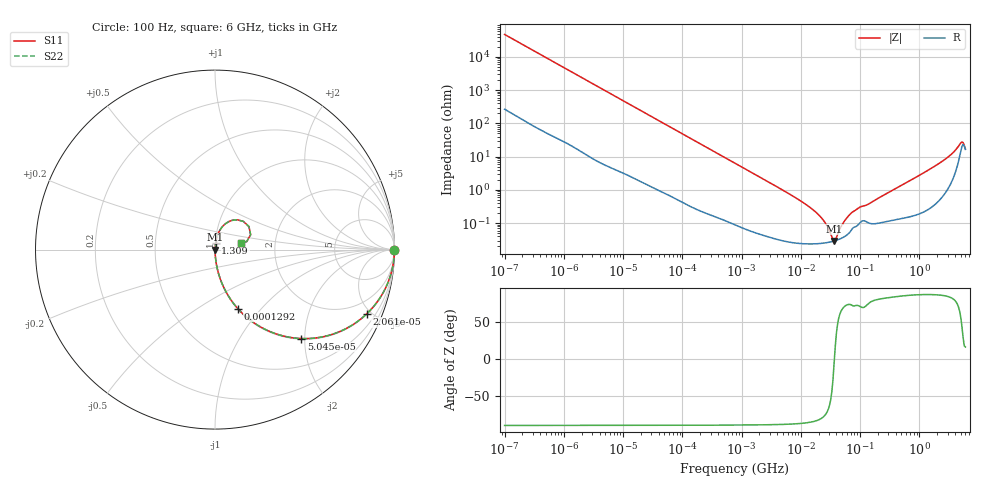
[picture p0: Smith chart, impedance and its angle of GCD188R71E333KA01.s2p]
!Murata Part Number: GCD188R71E333KA01
!These Parameters are Measured in Series Mode Connection
!Data Generated on Mar 13, 2026
!  o--ll--o
!Port1  Port2
!  o------o
!Operation Temp=25[degC], DC Bias Voltage=0[V]
!Freq. Start=100[Hz] Stop=6[GHz] 401[Steps]
# Hz S RI R 50
!Freq.(Hz) S11(Real) S11(Imag) S21(Real) S21(Imag) S12(Real) S12(Imag) S22(Real) S22(Imag)
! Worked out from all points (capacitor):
!   401 points, 100 Hz to 6 GHz, reference 50 ohm
!   read as one part in series: C = 33.5 nF near 109 Hz
!   lowest |Z| = 29.4 mohm at 36.42 MHz (marker M1)
!   series resonance near 36.95 MHz, so ESL is about 550 pH
!   S11 on the Smith chart (normalised r, x): 100 Hz: open; 20.61 kHz: 1.03, -4.69; 50.45 kHz: 1.02, -1.92; 129.2 kHz: 1.01, -0.75; 1.309 GHz: 1.00, +0.07; 6 GHz: 1.33, +0.09
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100  1 -0.00211  1.64e-05 0.00211  1.64e-05 0.00211  1 -0.00211
2008  0.998 -0.0418  0.002 0.0418  0.002 0.0418  0.998 -0.0418
7036  0.9782 -0.143  0.0218 0.143  0.0218 0.143  0.9782 -0.143
20606  0.8443 -0.359  0.1557 0.359  0.1557 0.359  0.8443 -0.359
40335  0.5901 -0.4878  0.4099 0.4878  0.4099 0.4878  0.5901 -0.4878
50455  0.4806 -0.4955  0.5194 0.4955  0.5194 0.4955  0.4806 -0.4955
129199  0.1269 -0.3284  0.8731 0.3284  0.8731 0.3284  0.1269 -0.3284
302498  0.0272 -0.1572  0.9728 0.1572  0.9728 0.1572  0.0272 -0.1572
774597  0.00491 -0.0633  0.9951 0.0633  0.9951 0.0633  0.00491 -0.0633
6353432  0.000329 -0.00764  0.9997 0.00764  0.9997 0.00764  0.000329 -0.00764
1.555665e7  0.000246 -0.00265  0.9998 0.00265  0.9998 0.00265  0.000246 -0.00265
2.434276e7  0.000254 -0.00117  0.9997 0.00117  0.9997 0.00117  0.000254 -0.00117
3.64232e7  0.000292 -3.82e-05  0.9997 3.82e-05  0.9997 3.82e-05  0.000292 -3.82e-05
3.983537e7  0.000307 0.000206  0.9997 -0.000206  0.9997 -0.000206  0.000307 0.000206
5.449875e7  0.000396 0.00109  0.9996 -0.00109  0.9996 -0.00109  0.000396 0.00109
7.129496e7  0.000621 0.00194  0.9994 -0.00194  0.9994 -0.00194  0.000621 0.00194
3.124326e8  0.00125 0.00859  0.9988 -0.00859  0.9988 -0.00859  0.00125 0.00859
1.309207e9  0.00368 0.0361  0.9963 -0.0361  0.9963 -0.0361  0.00368 0.0361
3.352442e9  0.0262 0.1064  0.9738 -0.1064  0.9738 -0.1064  0.0262 0.1064
4.796499e9  0.1244 0.1661  0.8756 -0.1661  0.8756 -0.1661  0.1244 0.1661
5.245841e9  0.189 0.1285  0.811 -0.1285  0.811 -0.1285  0.189 0.1285
6e9  0.1437 0.0344  0.8563 -0.0344  0.8563 -0.0344  0.1437 0.0344
